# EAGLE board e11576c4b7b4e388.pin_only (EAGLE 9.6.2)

Size 69.45 x 20.24 mm. Coordinates in mm from the lower left corner, seen from the top.
Outline: 0,0 69.45,0 69.45,20.24 0,20.24 0,0
Copper layers (1*16): Top 0.035mm / dielectric 1.5mm / Bottom 0.035mm
Design rules "default *": minimum track width 12mil, minimum drill 19mil, track to track 10mil, track to pad 10mil, pad to pad 10mil, via to via 10mil, smd to smd 10mil, copper to edge 10mil, drill to drill 8mil, minimum pad ring 10mil, minimum via ring 8mil, stop-mask expansion 4mil, vias tented up to drill 20mil, thermal gap 10mil
Holes 2.2 mm at 62.23,8.6 2.41,17.74 2.66,2.5

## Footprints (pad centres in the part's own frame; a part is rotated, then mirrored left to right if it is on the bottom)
C0805K = smd 1.1 x 1.4: 1 -1,0; 2 1,0
B/3528-21R = smd 1.95 x 2.5: + 1.525,0; - -1.525,0
CHIPLED_0805 = smd 1.2 x 1.2: A 0,-1.05; C 0,1.05
DIL28/3 = drill 0.813 pad 1.6 octagon: 1 -16.51,-3.81; 2 -13.97,-3.81; 3 -11.43,-3.81; 4 -8.89,-3.81; 5 -6.35,-3.81; 6 -3.81,-3.81; 7 -1.27,-3.81; 8 1.27,-3.81; 9 3.81,-3.81; 10 6.35,-3.81; 11 8.89,-3.81; 12 11.43,-3.81; 13 13.97,-3.81; 14 16.51,-3.81; 15 16.51,3.81; 16 13.97,3.81; 17 11.43,3.81; 18 8.89,3.81; 19 6.35,3.81; 20 3.81,3.81; 21 1.27,3.81; 22 -1.27,3.81; 23 -3.81,3.81; 24 -6.35,3.81; 25 -8.89,3.81; 26 -11.43,3.81; 27 -13.97,3.81; 28 -16.51,3.81
TSSOP28 = smd 0.35 x 1.2: 1 -4.225,-3.7; 2 -3.575,-3.7; 3 -2.925,-3.7; 4 -2.275,-3.7; 5 -1.625,-3.7; 6 -0.975,-3.7; 7 -0.325,-3.7; 8 0.325,-3.7; 9 0.975,-3.7; 10 1.625,-3.7; 11 2.275,-3.7; 12 2.925,-3.7; 13 3.575,-3.7; 14 4.225,-3.7; 15 4.225,3.7; 16 3.575,3.7; 17 2.925,3.7; 18 2.275,3.7; 19 1.625,3.7; 20 0.975,3.7; 21 0.325,3.7; 22 -0.325,3.7; 23 -0.975,3.7; 24 -1.625,3.7; 25 -2.275,3.7; 26 -2.925,3.7; 27 -3.575,3.7; 28 -4.225,3.7
1X06-CLEANBIG = drill 1.016 pad 1.778 octagon: 1 -6.35,0; 2 -3.81,0; 3 -1.27,0; 4 1.27,0; 5 3.81,0; 6 6.35,0
1X08-CLEANBIG = drill 1.016 pad 1.778 octagon: 1 -8.89,0; 2 -6.35,0; 3 -3.81,0; 4 -1.27,0; 5 1.27,0; 6 3.81,0; 7 6.35,0; 8 8.89,0
2X03 = drill 1.016 pad 1.676 octagon: 1 -2.54,-1.27; 2 -2.54,1.27; 3 0,-1.27; 4 0,1.27; 5 2.54,-1.27; 6 2.54,1.27
1X04-CB = drill 1.016 pad 1.676 octagon: 1 -3.81,0; 2 -1.27,0; 3 1.27,0; 4 3.81,0
1206 = smd 1.6 x 1.8: 1 -1.4,0; 2 1.4,0
R0805 = smd 1.1 x 1.4: 1 -1,0; 2 1,0
EVQ-Q2 = smd 3.2 x 1.2: A -3.4,-2; A' 3.4,-2; B -3.4,2; B' 3.4,2
SOLDERJUMPER_REFLOW = smd 1.168 x 1.6: 1 -0.762,0; 2 0.762,0
FIDUCIAL_1MM = smd 1 x 1: 1 0,0
USB-MINIB = smd 0.5 x 2.308: D+ 0,4.064; D- -0.8,4.064; GND 1.6,4.064; ID 0.8,4.064; VBUS -1.6,4.064 | smd 2 x 2.4: GND1 -4.4,-2; GND2 -4.4,3.5; GND3 4.4,3.5; GND4 4.4,-2 | hole 0.9: -2.2,1; 2.2,1
NX5032 = smd 2 x 2.4: P$1 2,0; P$2 -2,0

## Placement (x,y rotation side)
C1  0.1uF  [C0805K]  27.3,15.46 0 top
C2  100/6VuF  [B/3528-21R]  23.11,12.92 270 top
C3  0.1uF  [C0805K]  23.11,7.96 270 top
C4  0.1uF  [C0805K]  56,15.71 0 top
C5  15pF  [C0805K]  51.94,15.96 180 top
C6  15pF  [C0805K]  41.27,15.84 0 top
D1  [CHIPLED_0805]  5.58,3.26 0 top
D2  Green  [CHIPLED_0805]  5.2,17.49 180 top
IC1  ATMEGA168P  [DIL28/3]  43.05,8.6 180 top
IC2  FT232R  [TSSOP28]  16.38,6.44 0 top
JA1  [1X06-CLEANBIG]  53.21,1.23 0 top
JD1  [1X08-CLEANBIG]  32.89,19.01 180 top
JD2  [1X08-CLEANBIG]  32.89,1.23 0 top
JP3  [2X03]  66.42,3.9 270 top
JP4  [1X04-CB]  55.75,19.01 0 top
L1  [1206]  12.95,18.12 0 top
R1  10K  [R0805]  60.07,15.71 180 top
R2  1.0 K  [R0805]  9.27,2.63 0 top
R3  1.0 K  [R0805]  8.12,18.12 180 top
R4  1K  [R0805]  36.19,15.46 180 top
R5  1.0 K  [R0805]  15.62,14.06 90 top
R6  1.0 K  [R0805]  17.65,14.06 90 top
RX  Green  [CHIPLED_0805]  19.43,18 180 top
S1  EVQQ2  [EVQ-Q2]  66.29,14.57 90 top
SJ1  [SOLDERJUMPER_REFLOW]  12.57,14.82 270 top
TX  Green  [CHIPLED_0805]  16.63,18 180 top
U$1  FIDUCIAL  [FIDUCIAL_1MM]  62.23,1.87 0 top
U$2  FIDUCIAL  [FIDUCIAL_1MM]  20.44,14.95 0 top
U$3  [ADAFRUIT200MIL]  22.85,4.28 90 top
USB  [USB-MINIB]  4.82,10.12 270 top
X1  [NX5032]  46.48,16.09 180 top

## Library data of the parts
C1-C6 D1 D2 R1-R6 RX S1 TX U$1-U$3 USB X1 = adafruit
IC1 = avr
IC2 = ft232
JA1 JD1 JD2 JP4 = carduino
JP3 = pinhead-ez
L1 SJ1 = microbuilder

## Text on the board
tPlace: Vcc | RX | d6 | d5 | d4 | d3 | d2 | tx | rx | gnd | 3v | TX | d7 | rset | PWR | RST | CC2.5-by-sa | d8 | d9 | 10 | 11 | 12 | 13 | gnd | aref | a0 | a1 | a2 | a3 | a4 | a5 | USB-Boarduino | v2.0
bPlace: www.ladyada.net/ | make/boarduino | Arduino-compatible design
